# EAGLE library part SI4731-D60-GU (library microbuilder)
Silicon Labs Si4731 AM/FM/SW/LW Radio Receiver -- SSOP Package
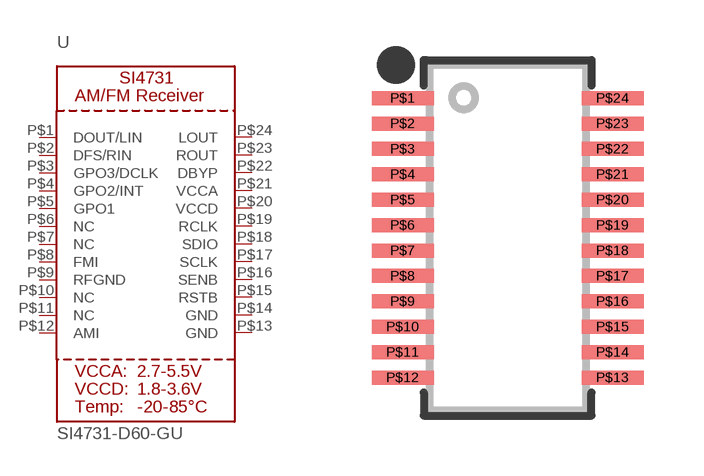
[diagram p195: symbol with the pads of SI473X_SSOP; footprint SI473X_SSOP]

Designator prefix U

## SI4731-D60-GU  [SI473X_SSOP]
P$1  DOUT/LIN
P$2  DFS/RIN
P$3  GPO3/DCLK
P$4  GPO2/INT
P$5  GPO1
P$6  NC
P$7  NC
P$8  FMI
P$9  RFGND
P$10  NC
P$11  NC
P$12  AMI
P$13  GND
P$14  GND
P$15  RSTB
P$16  SENB
P$17  SCLK
P$18  SDIO
P$19  RCLK
P$20  VCCD
P$21  VCCA
P$22  DBYP
P$23  ROUT
P$24  LOUT

## Footprint SI473X_SSOP (pad centres in mm)
Source: http://www.silabs.com/Support%20Documents/TechnicalDocs/Si4730-31-34-35-D60.pdf
smd 1.55 x 0.35: P$1 -2.625,3.493; P$2 -2.625,2.857; P$3 -2.625,2.223; P$4 -2.625,1.587; P$5 -2.625,0.953; P$6 -2.625,0.318; P$7 -2.625,-0.318; P$8 -2.625,-0.953; P$9 -2.625,-1.587; P$10 -2.625,-2.223; P$11 -2.625,-2.857; P$12 -2.625,-3.493; P$13 2.625,-3.493; P$14 2.625,-2.857; P$15 2.625,-2.223; P$16 2.625,-1.587; P$17 2.625,-0.953; P$18 2.625,-0.318; P$19 2.625,0.318; P$20 2.625,0.953; P$21 2.625,1.587; P$22 2.625,2.223; P$23 2.625,2.857; P$24 2.625,3.493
